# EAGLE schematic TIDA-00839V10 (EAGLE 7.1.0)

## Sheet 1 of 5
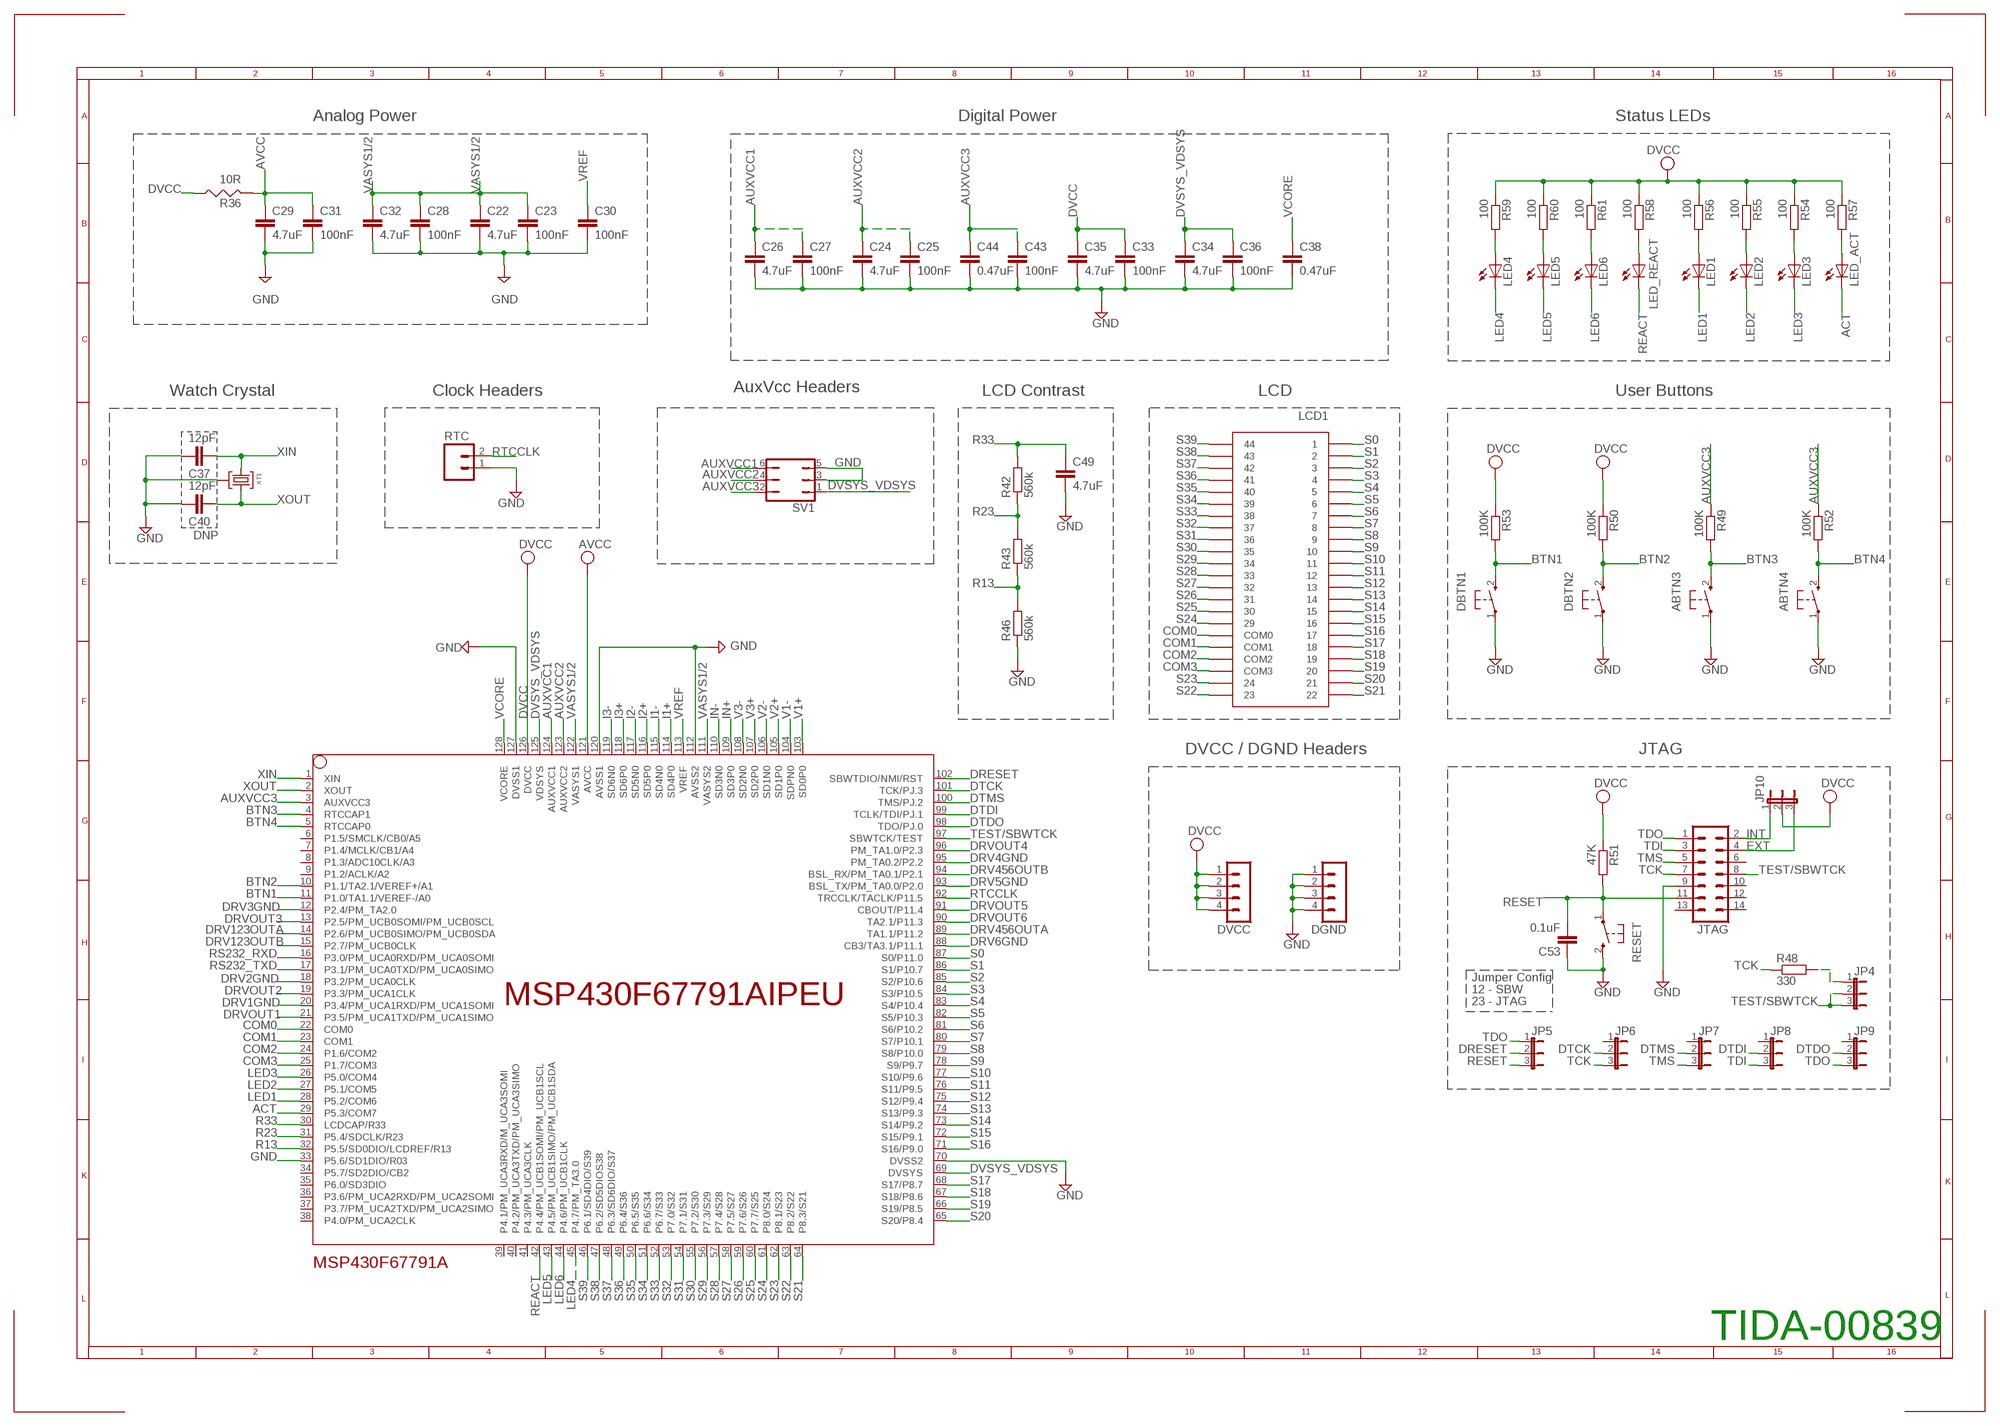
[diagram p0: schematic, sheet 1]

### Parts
ABTN3  PB  [PBTH]
ABTN4  PB  [PBTH]
C22  4.7uF  C-EUC0603  [C0603]
C23  100nF  C-EUC0603  [C0603]
C24  4.7uF  C-EUC0603  [C0603]
C25  100nF  C-EUC0603  [C0603]
C26  4.7uF  C-EUC0603  [C0603]
C27  100nF  C-EUC0603  [C0603]
C28  100nF  C-EUC0603  [C0603]
C29  4.7uF  C-EUC0603  [C0603]
C30  100nF  C-EUC0603  [C0603]
C31  100nF  C-EUC0603  [C0603]
C32  4.7uF  C-EUC0603  [C0603]
C33  100nF  C-EUC0603  [C0603]
C34  4.7uF  C-EUC0603  [C0603]
C35  4.7uF  C-EUC0603  [C0603]
C36  100nF  C-EUC0603  [C0603]
C37  12pF  C-EUC0603  [C0603]
C38  0.47uF  C-EUC0603  [C0603]
C40  12pF  C-EUC0603  [C0603]
C43  100nF  C-EUC0603  [C0603]
C44  0.47uF  C-EUC0603  [C0603]
C49  4.7uF  C-EUC0603  [C0603]
C53  0.1uF  C-EUC0603  [C0603]
DBTN1  PB  [PBTH]
DBTN2  PB  [PBTH]
DGND  MA04-1  [MA04-1]
DVCC  MA04-1  [MA04-1]
JP4  JP2E  [JP2]
JP5  JP2E  [JP2]
JP6  JP2E  [JP2]
JP7  JP2E  [JP2]
JP8  JP2E  [JP2]
JP9  JP2E  [JP2]
JP10  JP2E  [JP2]
JTAG  ML14  [ML14]
LCD1  TI_160SEG_LCD  [TI_160SEG_LCD]
LED1  LED3MM  [LED3MM]
LED2  LED3MM  [LED3MM]
LED3  LED3MM  [LED3MM]
LED4  LED3MM  [LED3MM]
LED5  LED3MM  [LED3MM]
LED6  LED3MM  [LED3MM]
LED_ACT  LED3MM  [LED3MM]
LED_REACT  LED3MM  [LED3MM]
MSP430F67791A  MSP430F6779AIPEU  [PEU128]
R36  10R  RES0805  [R0805]
R42  560k  R-EU_R0603  [R0603]
R43  560k  R-EU_R0603  [R0603]
R46  560k  R-EU_R0603  [R0603]
R48  330  R-EU_R0603  [R0603]
R49  100K  R-EU_R0603  [R0603]
R50  100K  R-EU_R0603  [R0603]
R51  47K  R-EU_R0603  [R0603]
R52  100K  R-EU_R0603  [R0603]
R53  100K  R-EU_R0603  [R0603]
R54  100  R-EU_R0603  [R0603]
R55  100  R-EU_R0603  [R0603]
R56  100  R-EU_R0603  [R0603]
R57  100  R-EU_R0603  [R0603]
R58  100  R-EU_R0603  [R0603]
R59  100  R-EU_R0603  [R0603]
R60  100  R-EU_R0603  [R0603]
R61  100  R-EU_R0603  [R0603]
RESET  PB  [PBTH]
RTC  M02PTH  [1X02]
SV1  JP3Q  [JP3Q]
XT1  CM200T  [CM200T]

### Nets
ACT: LED_ACT.K(C) MSP430F67791A.29(P5.3/COM7) ; also sheet 4
AUXVCC1: C26.1 C27.1 MSP430F67791A.124(AUXVCC1) SV1.6 ; also sheet 5
AUXVCC2: C24.1 C25.1 MSP430F67791A.123(AUXVCC2) SV1.4
AUXVCC3: C43.1 C44.1 MSP430F67791A.3(AUXVCC3) R49.1 R52.1 SV1.2
AVCC: C29.1 C31.1 MSP430F67791A.121(AVCC) R36.2 ; also sheet 2
BTN1: DBTN1.2(S) MSP430F67791A.11(P1.0/TA1.1/VEREF-/A0) R53.2
BTN2: DBTN2.2(S) MSP430F67791A.10(P1.1/TA2.1/VEREF+/A1) R50.2
BTN3: ABTN3.2(S) MSP430F67791A.4(RTCCAP1) R49.2
BTN4: ABTN4.2(S) MSP430F67791A.5(RTCCAP0) R52.2
COM0: LCD1.COM0 MSP430F67791A.22(COM0)
COM1: LCD1.COM1 MSP430F67791A.23(COM1)
COM2: LCD1.COM2 MSP430F67791A.24(P1.6/COM2)
COM3: LCD1.COM3 MSP430F67791A.25(P1.7/COM3)
DRESET: JP5.2 MSP430F67791A.102(SBWTDIO/NMI/RST)
DRV1GND: MSP430F67791A.20(P3.4/PM_UCA1RXD/PM_UCA1SOMI) ; also sheet 5
DRV2GND: MSP430F67791A.18(P3.2/PM_UCA0CLK) ; also sheet 5
DRV3GND: MSP430F67791A.12(P2.4/PM_TA2.0) ; also sheet 5
DRV4GND: MSP430F67791A.95(PM_TA0.2/P2.2) ; also sheet 5
DRV5GND: MSP430F67791A.93(BSL_TX/PM_TA0.0/P2.0) ; also sheet 5
DRV6GND: MSP430F67791A.88(CB3/TA3.1/P11.1) ; also sheet 5
DRV123OUTA: MSP430F67791A.14(P2.6/PM_UCB0SIMO/PM_UCB0SDA) ; also sheet 5
DRV123OUTB: MSP430F67791A.15(P2.7/PM_UCB0CLK) ; also sheet 5
DRV456OUTA: MSP430F67791A.89(TA1.1/P11.2) ; also sheet 5
DRV456OUTB: MSP430F67791A.94(BSL_RX/PM_TA0.1/P2.1) ; also sheet 5
DRVOUT1: MSP430F67791A.21(P3.5/PM_UCA1TXD/PM_UCA1SIMO) ; also sheet 5
DRVOUT2: MSP430F67791A.19(P3.3/PM_UCA1CLK) ; also sheet 5
DRVOUT3: MSP430F67791A.13(P2.5/PM_UCB0SOMI/PM_UCB0SCL) ; also sheet 5
DRVOUT4: MSP430F67791A.96(PM_TA1.0/P2.3) ; also sheet 5
DRVOUT5: MSP430F67791A.91(CBOUT/P11.4) ; also sheet 5
DRVOUT6: MSP430F67791A.90(TA2.1/P11.3) ; also sheet 5
DTCK: JP6.2 MSP430F67791A.101(TCK/PJ.3)
DTDI: JP8.2 MSP430F67791A.99(TCLK/TDI/PJ.1)
DTDO: JP9.2 MSP430F67791A.98(TDO/PJ.0)
DTMS: JP7.2 MSP430F67791A.100(TMS/PJ.2)
DVCC: C33.1 C35.1 DVCC.1 DVCC.2 DVCC.3 DVCC.4 JP10.2 MSP430F67791A.126(DVCC) R36.1 R50.1 R51.1 R53.1 R54.1 R55.1 R56.1 R57.1 R58.1 R59.1 R60.1 R61.1 ; also sheet 3,4,5
DVSYS_VDSYS: C34.1 C36.1 MSP430F67791A.69(DVSYS) MSP430F67791A.125(VDSYS) SV1.1 ; also sheet 5
EXT: JP10.3 JTAG.4
GND: ABTN3.1(P) ABTN4.1(P) C22.2 C23.2 C24.2 C25.2 C26.2 C27.2 C28.2 C29.2 C30.2 C31.2 C32.2 C33.2 C34.2 C35.2 C36.2 C37.2 C38.2 C40.2 C43.2 C44.2 C49.2 C53.1 DBTN1.1(P) DBTN2.1(P) DGND.1 DGND.2 DGND.3 DGND.4 JTAG.9 MSP430F67791A.33(P5.6/SD1DIO/R03) MSP430F67791A.70(DVSS2) MSP430F67791A.112(AVSS2) MSP430F67791A.120(AVSS1) MSP430F67791A.127(DVSS1) R46.1 RESET.2(S) RTC.1 SV1.3 SV1.5 XT1.P3 ; also sheet 2,3,4,5
I1+: MSP430F67791A.114(SD4P0) ; also sheet 2
I1-: MSP430F67791A.115(SD4N0) ; also sheet 2
I2+: MSP430F67791A.116(SD5P0) ; also sheet 2
I2-: MSP430F67791A.117(SD5N0) ; also sheet 2
I3+: MSP430F67791A.118(SD6P0) ; also sheet 2
I3-: MSP430F67791A.119(SD6N0) ; also sheet 2
IN+: MSP430F67791A.109(SD3P0) ; also sheet 2
IN-: MSP430F67791A.110(SD3N0) ; also sheet 2
INT: JP10.1 JTAG.2
LED1: LED1.K(C) MSP430F67791A.28(P5.2/COM6)
LED2: LED2.K(C) MSP430F67791A.27(P5.1/COM5)
LED3: LED3.K(C) MSP430F67791A.26(P5.0/COM4)
LED4: LED4.K(C) MSP430F67791A.45(P4.7/PM_TA3.0)
LED5: LED5.K(C) MSP430F67791A.43(P4.5/PM_UCB1SIMO/PM_UCB1SDA)
LED6: LED6.K(C) MSP430F67791A.44(P4.6/PM_UCB1CLK)
N$4: LED1.A R56.2
N$7: LED2.A R55.2
N$10: JP4.1 R48.2
N$21: LED4.A R59.2
N$27: LED5.A R60.2
N$30: LED3.A R54.2
N$36: LED6.A R61.2
N$44: LED_REACT.A R58.2
N$46: LED_ACT.A R57.2
R13: MSP430F67791A.32(P5.5/SD0DIO/LCDREF/R13) R43.1 R46.2
R23: MSP430F67791A.31(P5.4/SDCLK/R23) R42.1 R43.2
R33: C49.1 MSP430F67791A.30(LCDCAP/R33) R42.2
REACT: LED_REACT.K(C) MSP430F67791A.42(P4.4/PM_UCB1SOMI/PM_UCB1SCL) ; also sheet 4
RESET: C53.2 JP5.3 JTAG.11 R51.2 RESET.1(P)
RS232_RXD: MSP430F67791A.16(P3.0/PM_UCA0RXD/PM_UCA0SOMI) ; also sheet 4
RS232_TXD: MSP430F67791A.17(P3.1/PM_UCA0TXD/PM_UCA0SIMO) ; also sheet 4
RTCCLK: MSP430F67791A.92(TRCCLK/TACLK/P11.5) RTC.2
S0: LCD1.1 MSP430F67791A.87(S0/P11.0)
S1: LCD1.2 MSP430F67791A.86(S1/P10.7)
S2: LCD1.3 MSP430F67791A.85(S2/P10.6)
S3: LCD1.4 MSP430F67791A.84(S3/P10.5)
S4: LCD1.5 MSP430F67791A.83(S4/P10.4)
S5: LCD1.6 MSP430F67791A.82(S5/P10.3)
S6: LCD1.7 MSP430F67791A.81(S6/P10.2)
S7: LCD1.8 MSP430F67791A.80(S7/P10.1)
S8: LCD1.9 MSP430F67791A.79(S8/P10.0)
S9: LCD1.10 MSP430F67791A.78(S9/P9.7)
S10: LCD1.11 MSP430F67791A.77(S10/P9.6)
S11: LCD1.12 MSP430F67791A.76(S11/P9.5)
S12: LCD1.13 MSP430F67791A.75(S12/P9.4)
S13: LCD1.14 MSP430F67791A.74(S13/P9.3)
S14: LCD1.15 MSP430F67791A.73(S14/P9.2)
S15: LCD1.16 MSP430F67791A.72(S15/P9.1)
S16: LCD1.17 MSP430F67791A.71(S16/P9.0)
S17: LCD1.18 MSP430F67791A.68(S17/P8.7)
S18: LCD1.19 MSP430F67791A.67(S18/P8.6)
S19: LCD1.20 MSP430F67791A.66(S19/P8.5)
S20: LCD1.21 MSP430F67791A.65(S20/P8.4)
S21: LCD1.22 MSP430F67791A.64(P8.3/S21)
S22: LCD1.23 MSP430F67791A.63(P8.2/S22)
S23: LCD1.24 MSP430F67791A.62(P8.1/S23)
S24: LCD1.29 MSP430F67791A.61(P8.0/S24)
S25: LCD1.30 MSP430F67791A.60(P7.7/S25)
S26: LCD1.31 MSP430F67791A.59(P7.6/S26)
S27: LCD1.32 MSP430F67791A.58(P7.5/S27)
S28: LCD1.33 MSP430F67791A.57(P7.4/S28)
S29: LCD1.34 MSP430F67791A.56(P7.3/S29)
S30: LCD1.35 MSP430F67791A.55(P7.2/S30)
S31: LCD1.36 MSP430F67791A.54(P7.1/S31)
S32: LCD1.37 MSP430F67791A.53(P7.0/S32)
S33: LCD1.38 MSP430F67791A.52(P6.7/S33)
S34: LCD1.39 MSP430F67791A.51(P6.6/S34)
S35: LCD1.40 MSP430F67791A.50(P6.5/S35)
S36: LCD1.41 MSP430F67791A.49(P6.4/S36)
S37: LCD1.42 MSP430F67791A.48(P6.3/SD6DIO/S37)
S38: LCD1.43 MSP430F67791A.47(P6.2/SD5DIOS38)
S39: LCD1.44 MSP430F67791A.46(P6.1/SD4DIO/S39)
TCK: JP6.3 JTAG.7 R48.1
TDI: JP8.3 JTAG.3
TDO: JP5.1 JP9.3 JTAG.1
TEST/SBWTCK: JP4.2 JP4.3 JTAG.8 MSP430F67791A.97(SBWTCK/TEST)
TMS: JP7.3 JTAG.5
V1+: MSP430F67791A.103(SD0P0) ; also sheet 2
V1-: MSP430F67791A.104(SDPN0) ; also sheet 2
V2+: MSP430F67791A.105(SD1P0) ; also sheet 2
V2-: MSP430F67791A.106(SD1N0) ; also sheet 2
V3+: MSP430F67791A.107(SD2P0) ; also sheet 2
V3-: MSP430F67791A.108(SD2N0) ; also sheet 2
VASYS1/2: C22.1 C23.1 C28.1 C32.1 MSP430F67791A.111(VASYS2) MSP430F67791A.122(VASYS1)
VCORE: C38.1 MSP430F67791A.128(VCORE)
VREF: C30.1 MSP430F67791A.113(VREF)
XIN: C37.1 MSP430F67791A.1(XIN) XT1.P2
XOUT: C40.1 MSP430F67791A.2(XOUT) XT1.P1
Unconnected: JP6.1 JP7.1 JP8.1 JP9.1 JTAG.6 JTAG.10 JTAG.12 JTAG.13 JTAG.14 MSP430F67791A.6(P1.5/SMCLK/CB0/A5) MSP430F67791A.7(P1.4/MCLK/CB1/A4) MSP430F67791A.8(P1.3/ADC10CLK/A3) MSP430F67791A.9(P1.2/ACLK/A2) MSP430F67791A.34(P5.7/SD2DIO/CB2) MSP430F67791A.35(P6.0/SD3DIO) MSP430F67791A.36(P3.6/PM_UCA2RXD/PM_UCA2SOMI) MSP430F67791A.37(P3.7/PM_UCA2TXD/PM_UCA2SIMO) MSP430F67791A.38(P4.0/PM_UCA2CLK) MSP430F67791A.39(P4.1/PM_UCA3RXD/M_UCA3SOMI) MSP430F67791A.40(P4.2/PM_UCA3TXD/PM_UCA3SIMO) MSP430F67791A.41(P4.3/PM_UCA3CLK)

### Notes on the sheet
- Analog Power | Digital Power | Status LEDs
- Watch Crystal | Clock Headers | AuxVcc Headers | LCD Contrast | LCD | User Buttons
- DNP
- DVCC / DGND Headers | JTAG
- Jumper Config
- 12 - SBW
- 23 - JTAG
- TIDA-00839

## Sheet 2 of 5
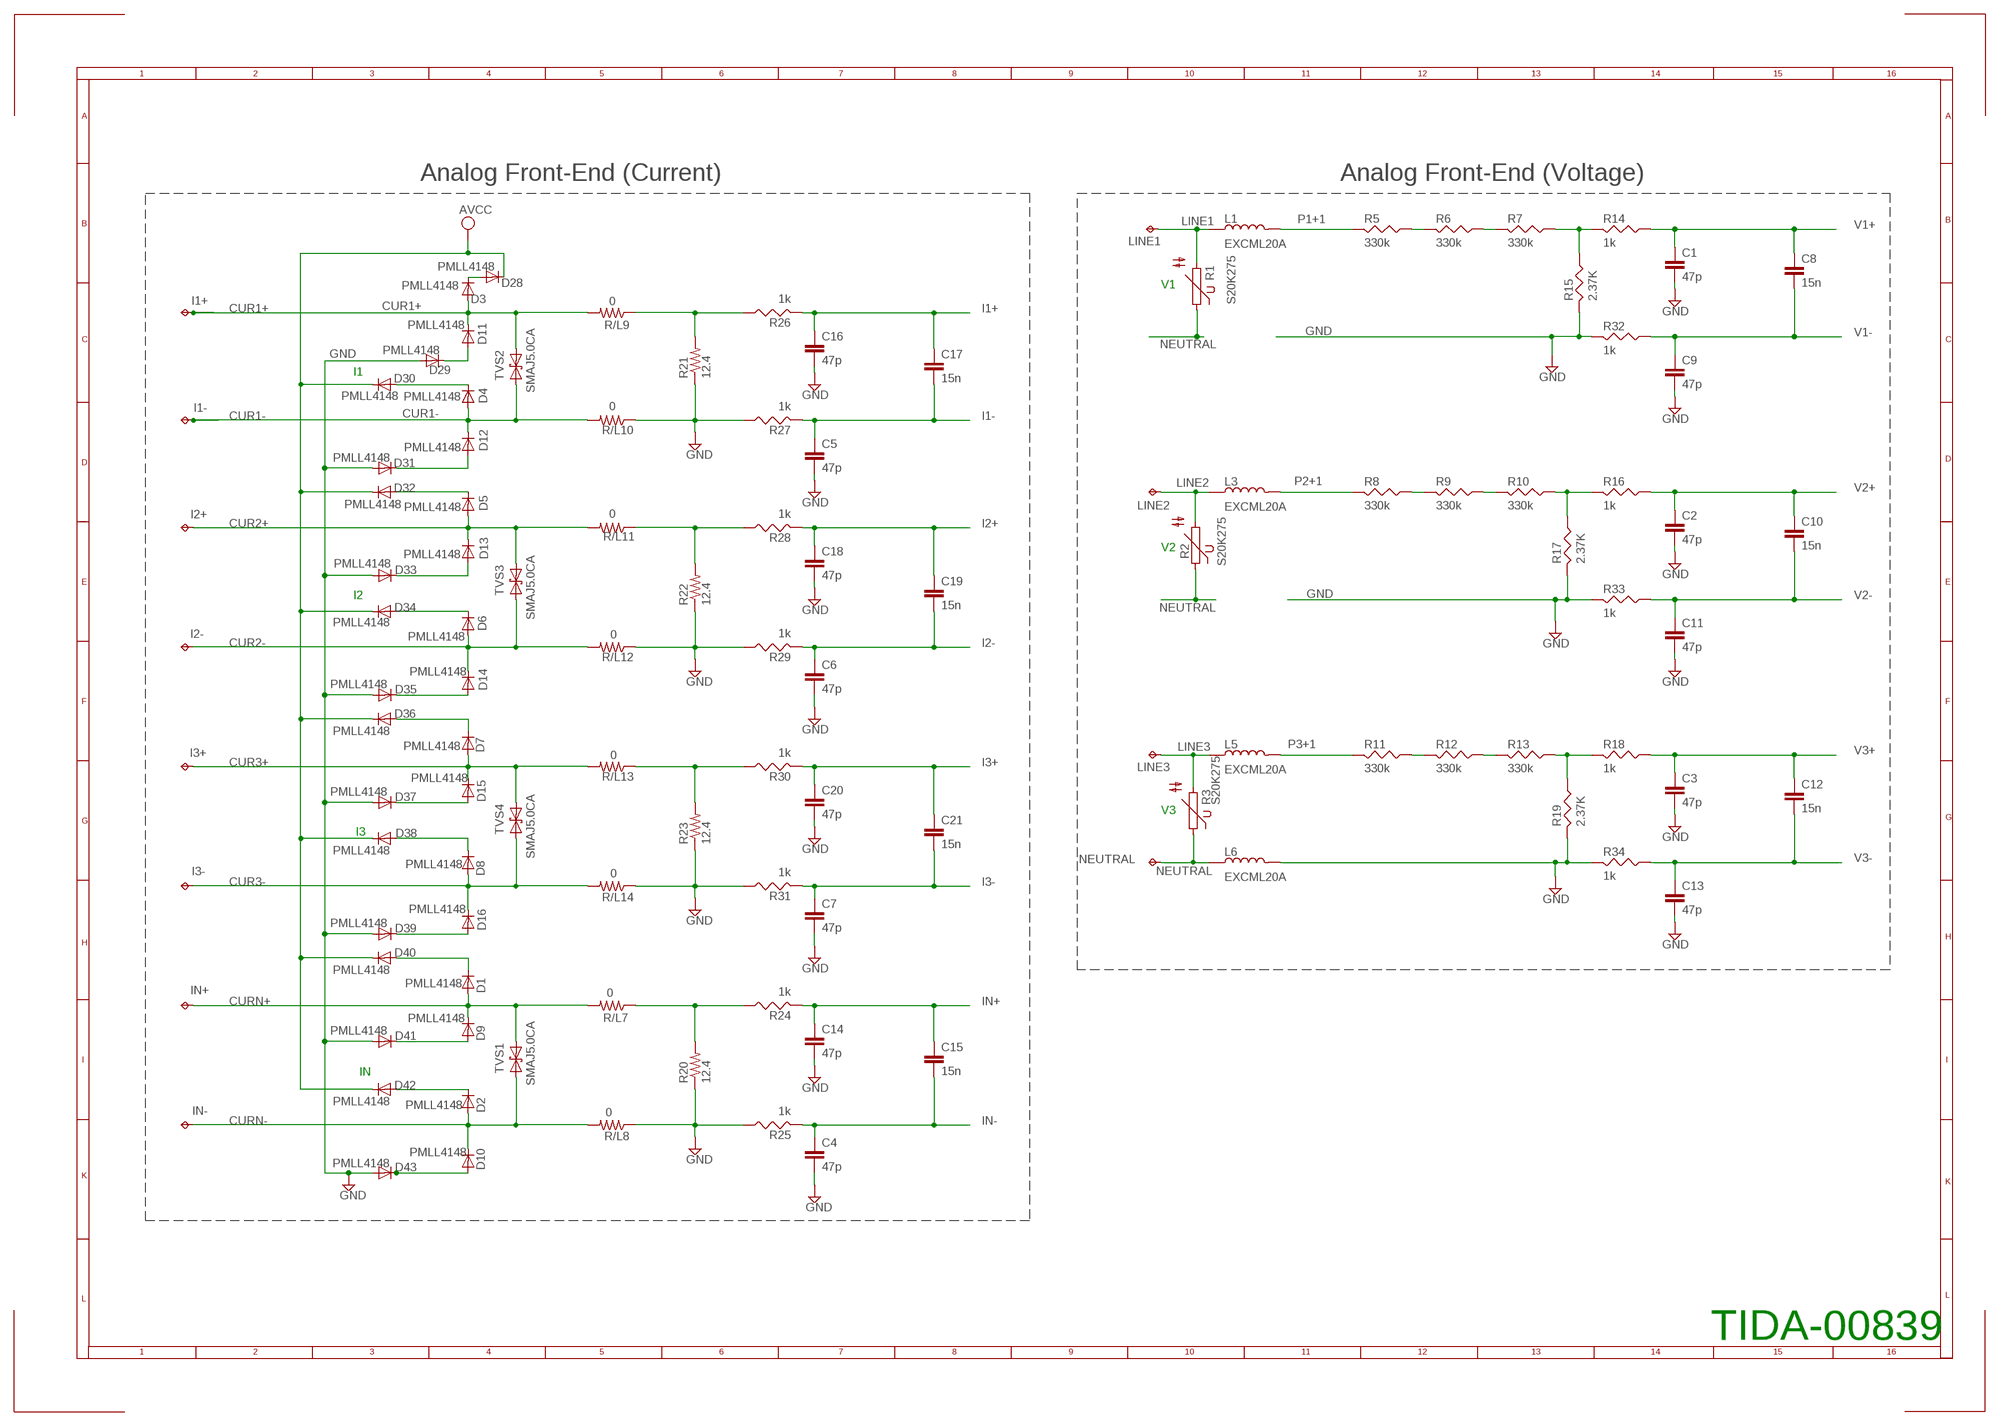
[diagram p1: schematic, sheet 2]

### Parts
C1  47p  C-EUC0805  [C0805]
C2  47p  C-EUC0805  [C0805]
C3  47p  C-EUC0805  [C0805]
C4  47p  C-EUC0805  [C0805]
C5  47p  C-EUC0805  [C0805]
C6  47p  C-EUC0805  [C0805]
C7  47p  C-EUC0805  [C0805]
C8  15n  C-EUC0805  [C0805]
C9  47p  C-EUC0805  [C0805]
C10  15n  C-EUC0805  [C0805]
C11  47p  C-EUC0805  [C0805]
C12  15n  C-EUC0805  [C0805]
C13  47p  C-EUC0805  [C0805]
C14  47p  C-EUC0805  [C0805]
C15  15n  C-EUC0805  [C0805]
C16  47p  C-EUC0805  [C0805]
C17  15n  C-EUC0805  [C0805]
C18  47p  C-EUC0805  [C0805]
C19  15n  C-EUC0805  [C0805]
C20  47p  C-EUC0805  [C0805]
C21  15n  C-EUC0805  [C0805]
D1  PMLL4148  [SOD80C]
D2  PMLL4148  [SOD80C]
D3  PMLL4148  [SOD80C]
D4  PMLL4148  [SOD80C]
D5  PMLL4148  [SOD80C]
D6  PMLL4148  [SOD80C]
D7  PMLL4148  [SOD80C]
D8  PMLL4148  [SOD80C]
D9  PMLL4148  [SOD80C]
D10  PMLL4148  [SOD80C]
D11  PMLL4148  [SOD80C]
D12  PMLL4148  [SOD80C]
D13  PMLL4148  [SOD80C]
D14  PMLL4148  [SOD80C]
D15  PMLL4148  [SOD80C]
D16  PMLL4148  [SOD80C]
D28  PMLL4148  [SOD80C]
D29  PMLL4148  [SOD80C]
D30  PMLL4148  [SOD80C]
D31  PMLL4148  [SOD80C]
D32  PMLL4148  [SOD80C]
D33  PMLL4148  [SOD80C]
D34  PMLL4148  [SOD80C]
D35  PMLL4148  [SOD80C]
D36  PMLL4148  [SOD80C]
D37  PMLL4148  [SOD80C]
D38  PMLL4148  [SOD80C]
D39  PMLL4148  [SOD80C]
D40  PMLL4148  [SOD80C]
D41  PMLL4148  [SOD80C]
D42  PMLL4148  [SOD80C]
D43  PMLL4148  [SOD80C]
I1+  TPPAD1-20  [P1-20]
I1-  TPPAD1-20  [P1-20]
I2+  TPPAD1-20  [P1-20]
I2-  TPPAD1-20  [P1-20]
I3+  TPPAD1-20  [P1-20]
I3-  TPPAD1-20  [P1-20]
IN+  TPPAD1-20  [P1-20]
IN-  TPPAD1-20  [P1-20]
L1  EXCML20A  EXCELSA390805  [R0805]
L3  EXCML20A  EXCELSA390805  [R0805]
L5  EXCML20A  EXCELSA390805  [R0805]
L6  EXCML20A  EXCELSA390805  [R0805]
LINE1  TPPAD1-20  [P1-20]
LINE2  TPPAD1-20  [P1-20]
LINE3  TPPAD1-20  [P1-20]
NEUTRAL  TPPAD1-20  [P1-20]
R1  S20K275  [S20K275]
R2  S20K275  [S20K275]
R3  S20K275  [S20K275]
R5  330k  RES0805  [R0805]
R6  330k  RES0805  [R0805]
R7  330k  RES0805  [R0805]
R8  330k  RES0805  [R0805]
R9  330k  RES0805  [R0805]
R10  330k  RES0805  [R0805]
R11  330k  RES0805  [R0805]
R12  330k  RES0805  [R0805]
R13  330k  RES0805  [R0805]
R14  1k  RES0805  [R0805]
R15  2.37K  RES0805  [R0805]
R16  1k  RES0805  [R0805]
R17  2.37K  RES0805  [R0805]
R18  1k  RES0805  [R0805]
R19  2.37K  RES0805  [R0805]
R20  12.4  R-US_R0805  [R0805]
R21  12.4  R-US_R0805  [R0805]
R22  12.4  R-US_R0805  [R0805]
R23  12.4  R-US_R0805  [R0805]
R24  1k  RES0805  [R0805]
R25  1k  RES0805  [R0805]
R26  1k  RES0805  [R0805]
R27  1k  RES0805  [R0805]
R28  1k  RES0805  [R0805]
R29  1k  RES0805  [R0805]
R30  1k  RES0805  [R0805]
R31  1k  RES0805  [R0805]
R32  1k  RES0805  [R0805]
R33  1k  RES0805  [R0805]
R34  1k  RES0805  [R0805]
R/L7  0  R-US_R0805  [R0805]
R/L8  0  R-US_R0805  [R0805]
R/L9  0  R-US_R0805  [R0805]
R/L10  0  R-US_R0805  [R0805]
R/L11  0  R-US_R0805  [R0805]
R/L12  0  R-US_R0805  [R0805]
R/L13  0  R-US_R0805  [R0805]
R/L14  0  R-US_R0805  [R0805]
TVS1  SMAJ5.0CA  [DO214AC]
TVS2  SMAJ5.0CA  [DO214AC]
TVS3  SMAJ5.0CA  [DO214AC]
TVS4  SMAJ5.0CA  [DO214AC]

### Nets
AVCC: D28.C D30.C D32.C D34.C D36.C D38.C D40.C D42.C ; also sheet 1
CUR1+: D3.A D11.C I1+.TP R/L9.2 TVS2.C(K)
CUR1-: D4.A D12.C I1-.TP R/L10.2 TVS2.A
CUR2+: D5.A D13.C I2+.TP R/L11.2 TVS3.C(K)
CUR2-: D6.A D14.C I2-.TP R/L12.2 TVS3.A
CUR3+: D7.A D15.C I3+.TP R/L13.2 TVS4.C(K)
CUR3-: D8.A D16.C I3-.TP R/L14.2 TVS4.A
CURN+: D1.A D9.C IN+.TP R/L7.2 TVS1.C(K)
CURN-: D2.A D10.C IN-.TP R/L8.2 TVS1.A
GND: C1.2 C2.2 C3.2 C4.2 C5.2 C6.2 C7.2 C9.2 C11.2 C13.2 C14.2 C16.2 C18.2 C20.2 D29.A D31.A D33.A D35.A D37.A D39.A D41.A D43.A L6.2 R15.2 R17.2 R19.2 R20.1 R21.1 R22.1 R23.1 R25.1 R27.1 R29.1 R31.1 R32.2 R33.2 R34.2 R/L8.1 R/L10.1 R/L12.1 R/L14.1 ; also sheet 1,3,4,5
I1+: C16.1 C17.1 R26.2 ; also sheet 1
I1-: C5.1 C17.2 R27.2 ; also sheet 1
I2+: C18.1 C19.1 R28.2 ; also sheet 1
I2-: C6.1 C19.2 R29.2 ; also sheet 1
I3+: C20.1 C21.1 R30.2 ; also sheet 1
I3-: C7.1 C21.2 R31.2 ; also sheet 1
IN+: C14.1 C15.1 R24.2 ; also sheet 1
IN-: C4.1 C15.2 R25.2 ; also sheet 1
LINE1: L1.1 LINE1.TP R1.2
LINE2: L3.1 LINE2.TP R2.2
LINE3: L5.1 LINE3.TP R3.2
N$6: R20.2 R24.1 R/L7.1
N$8: R5.1 R6.2
N$13: R6.1 R7.2
N$14: R7.1 R14.2 R15.1
N$15: R8.1 R9.2
N$16: R9.1 R10.2
N$19: R10.1 R16.2 R17.1
N$20: D3.C D28.A
N$23: D11.A D29.C
N$25: R23.2 R30.1 R/L13.1
N$29: R11.1 R12.2
N$31: R22.2 R28.1 R/L11.1
N$32: R21.2 R26.1 R/L9.1
N$33: R12.1 R13.2
N$34: R13.1 R18.2 R19.1
N$39: D4.C D30.A
N$40: D12.A D31.C
N$42: D5.C D32.A
N$54: D13.A D33.C
N$62: D6.C D34.A
N$63: D14.A D35.C
N$64: D7.C D36.A
N$66: D15.A D37.C
N$70: D8.C D38.A
N$73: D16.A D39.C
N$74: D1.C D40.A
N$75: D9.A D41.C
N$76: D2.C D42.A
N$77: D10.A D43.C
NEUTRAL: L6.1 NEUTRAL.TP R1.1 R2.1 R3.1 ; also sheet 3
P1+1: L1.2 R5.2 ; also sheet 3
P2+1: L3.2 R8.2 ; also sheet 3
P3+1: L5.2 R11.2 ; also sheet 3
V1+: C1.1 C8.1 R14.1 ; also sheet 1
V1-: C8.2 C9.1 R32.1 ; also sheet 1
V2+: C2.1 C10.1 R16.1 ; also sheet 1
V2-: C10.2 C11.1 R33.1 ; also sheet 1
V3+: C3.1 C12.1 R18.1 ; also sheet 1
V3-: C12.2 C13.1 R34.1 ; also sheet 1

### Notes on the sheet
- Analog Front-End (Current) | Analog Front-End (Voltage)
- V1
- I1
- V2
- I2
- V3
- I3
- IN
- TIDA-00839

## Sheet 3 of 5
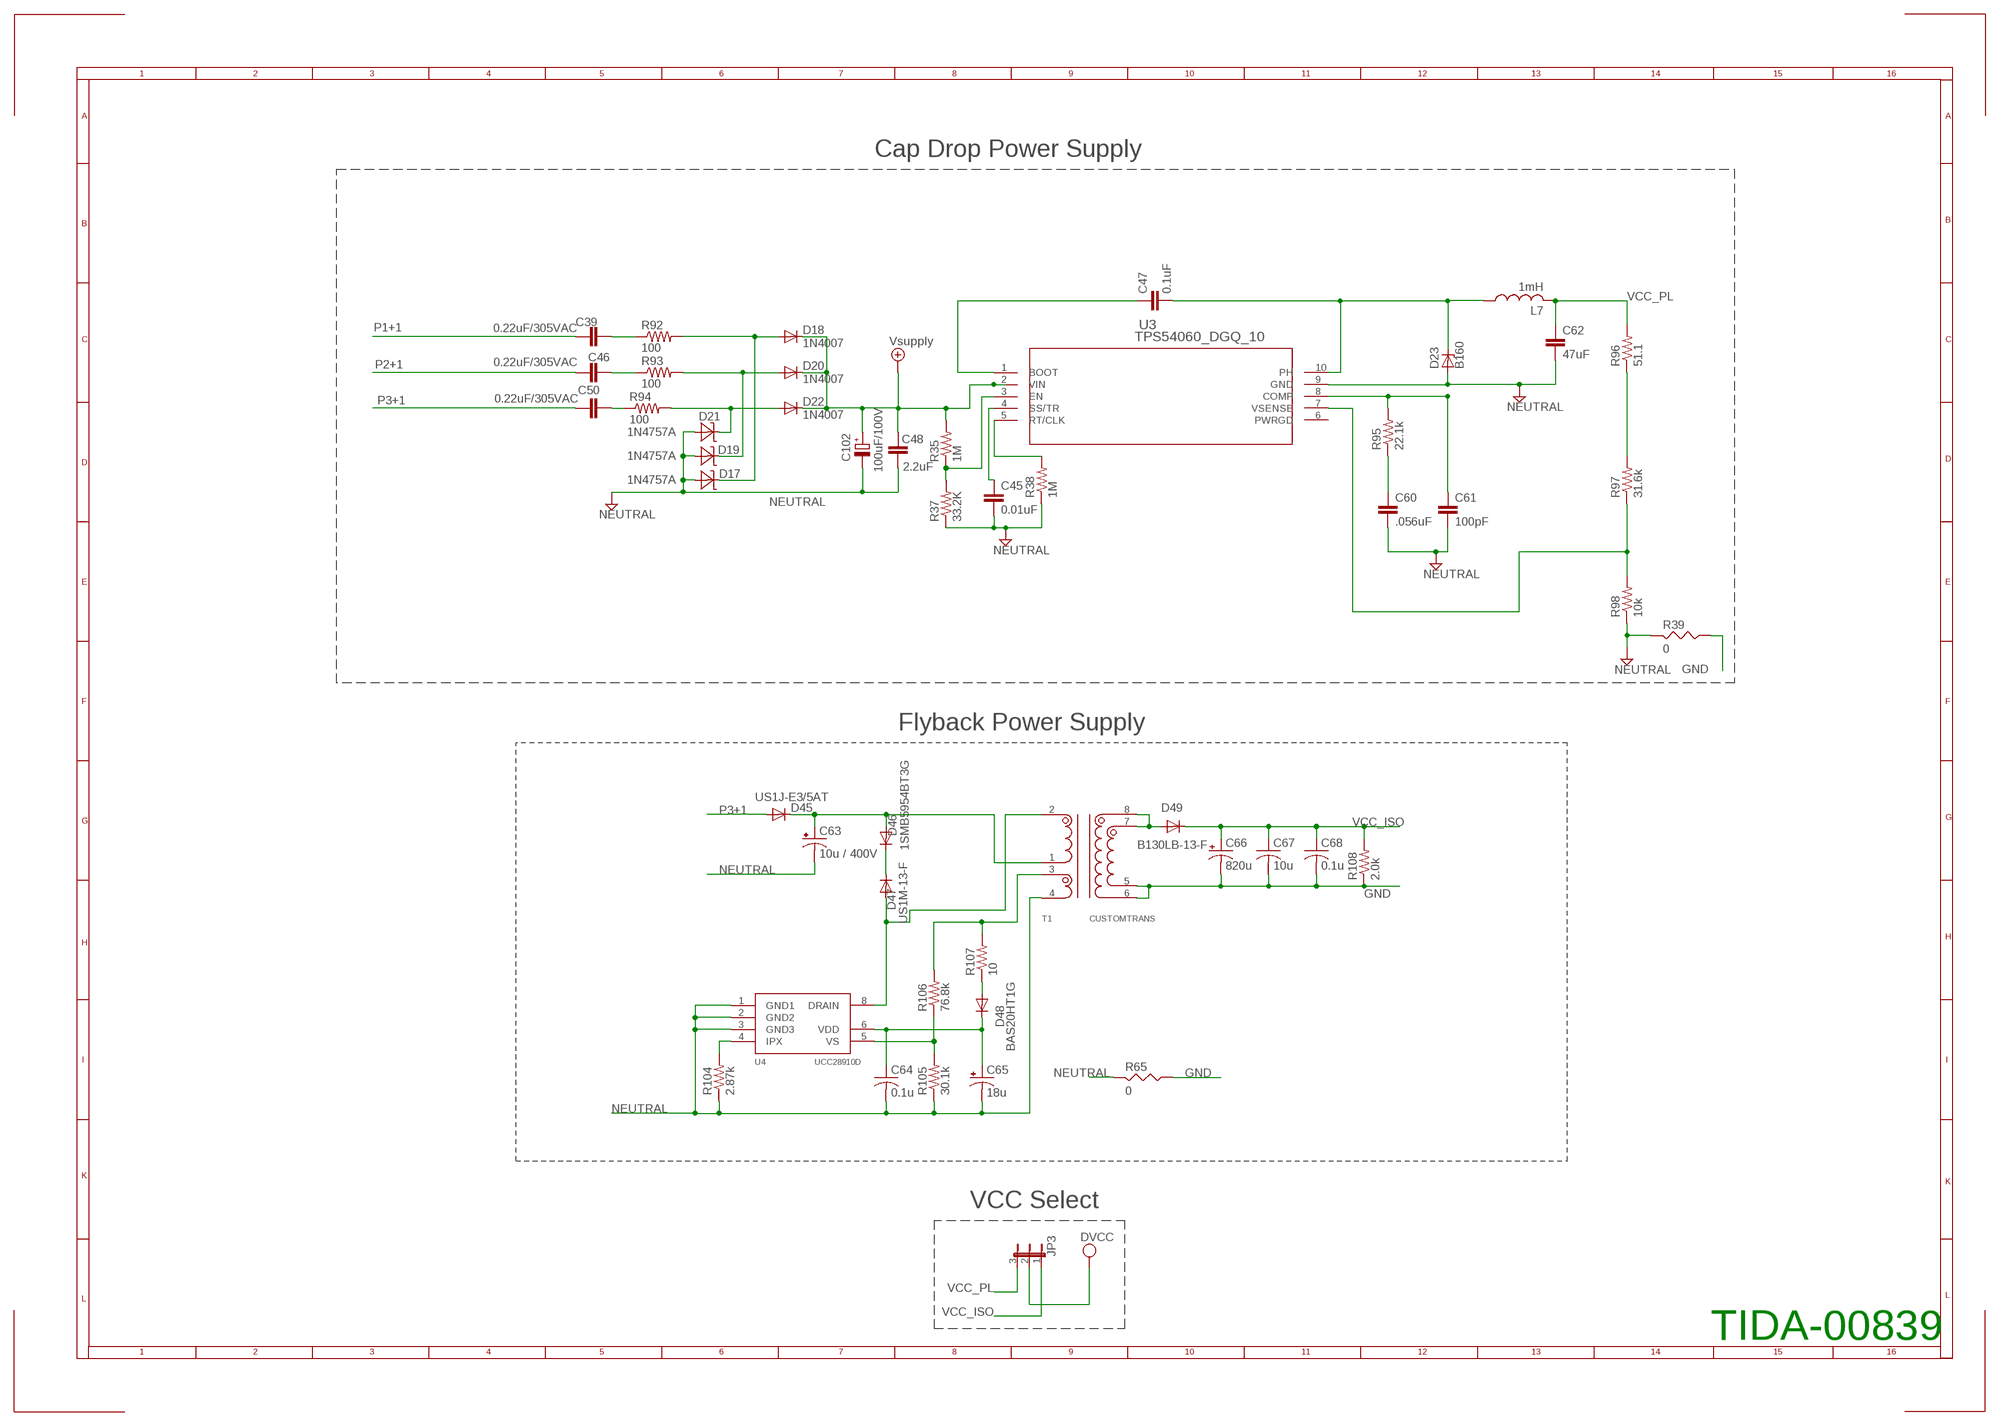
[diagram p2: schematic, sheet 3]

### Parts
C39  0.22uF/305VAC  C15/8  [C15B8]
C45  0.01uF  C-EUC0603  [C0603]
C46  0.22uF/305VAC  C15/8  [C15B8]
C47  0.1uF  C-EUC0603  [C0603]
C48  2.2uF  C-EUC1210  [C1210]
C50  0.22uF/305VAC  C15/8  [C15B8]
C60  .056uF  C-EUC0603  [C0603]
C61  100pF  C-EUC0603  [C0603]
C62  47uF  C-EUC1210  [C1210]
C63  10u / 400V  CPOL-USE5-10.5  [E5-10,5]
C64  0.1u  C-USC0603  [C0603]
C65  18u  CPOL-USE5-5  [E5-5]
C66  820u  CPOL-USE3.5-8  [E3,5-8]
C67  10u  C-USC1210  [C1210]
C68  0.1u  C-USC0805  [C0805]
C102  100uF/100V  CPOL-EUE5-10.5  [E5-10,5]
D17  1N4757A  [DO41Z10]
D18  1N4007  [DO41-10]
D19  1N4757A  [DO41Z10]
D20  1N4007  [DO41-10]
D21  1N4757A  [DO41Z10]
D22  1N4007  [DO41-10]
D23  B160  ZENER-DIODESMB  [SMB]
D45  US1J-E3/5AT  DIODE-DO-214AC  [DO-214AC]
D46  1SMB5954BT3G  DIODE-DO-214AC  [DO-214AC]
D47  US1M-13-F  DIODE-DO-214AC  [DO-214AC]
D48  BAS20HT1G  DIODE-SOD323-R  [SOD323-R]
D49  B130LB-13-F  DIODE-DO214AA  [DO214AA]
JP3  JP2E  [JP2]
L7  1mH  L-USMSS1038-105  [INDUCTOR_POWER_SUPPLY_6779]
R35  1M  R-US_R0603  [R0603]
R37  33.2K  R-US_R0603  [R0603]
R38  1M  R-US_R0603  [R0603]
R39  0  RES0805  [R0805]
R65  0  RES0805  [R0805]
R92  100  R-US_0414/15  [0414/15]
R93  100  R-US_0414/15  [0414/15]
R94  100  R-US_0414/15  [0414/15]
R95  22.1k  R-US_R0603  [R0603]
R96  51.1  R-US_R0603  [R0603]
R97  31.6k  R-US_R0603  [R0603]
R98  10k  R-US_R0603  [R0603]
R104  2.87k  R-US_R0603  [R0603]
R105  30.1k  R-US_R0603  [R0603]
R106  76.8k  R-US_R0603  [R0603]
R107  10  R-US_R0603  [R0603]
R108  2.0k  R-US_R0603  [R0603]
T1  CUSTOMTRANS  [TRANS]
U3  TPS54060_DGQ_10  [DGQ10_1P88X1P57]
U4  UCC28910D  [SOIC(D)]

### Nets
DVCC: JP3.2 ; also sheet 1,4,5
GND: C66.- C67.2 C68.2 R39.1 R65.1 R108.1 T1.5 T1.6 ; also sheet 1,2,4,5
N$17: R38.2 U3.5(RT/CLK)
N$18: D17.C D18.A R92.2
N$37: C45.1 U3.4(SS/TR)
N$38: R35.1 R37.2 U3.3(EN)
N$47: D19.C D20.A R93.2
N$78: C47.1 U3.1(BOOT)
N$80: C47.2 D23.C L7.1 U3.10(PH)
N$82: C60.1 R95.1
N$84: C39.2 R92.1
N$89: C46.2 R93.1
N$90: C50.2 R94.1
N$91: C63.+ D45.C D46.A T1.1
N$92: C61.1 R95.2 U3.8(COMP)
N$93: R96.1 R97.2
N$94: D21.C D22.A R94.2
N$95: R97.1 R98.2 U3.7(VSENSE)
N$96: D46.C D47.C
N$97: R104.2 U4.4(IPX)
N$98: D47.A T1.2 U4.8(DRAIN)
N$99: C64.1 C65.+ D48.C U4.6(VDD)
N$100: R105.2 R106.1 U4.5(VS)
N$101: D48.A R107.1
N$102: R106.2 R107.2 T1.3
N$103: D49.A T1.7 T1.8
NEUTRAL: C45.2 C48.2 C60.2 C61.2 C62.2 C63.- C64.2 C65.- C102.- D17.A D19.A D21.A D23.A R37.1 R38.1 R39.2 R65.2 R98.1 R104.1 R105.1 T1.4 U3.9(GND) U4.1(GND1) U4.2(GND2) U4.3(GND3) ; also sheet 2
P1+1: C39.1 ; also sheet 2
P2+1: C46.1 ; also sheet 2
P3+1: C50.1 D45.A ; also sheet 2
VCC_ISO: C66.+ C67.1 C68.1 D49.C JP3.1 R108.2
VCC_PL: C62.1 JP3.3 L7.2 R96.2
VSUPPLY: C48.1 C102.+ D18.C D20.C D22.C R35.2 U3.2(VIN) ; supply symbol labelled Vsupply
Unconnected: U3.6(PWRGD)

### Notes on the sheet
- Cap Drop Power Supply
- Flyback Power Supply
- VCC Select
- TIDA-00839

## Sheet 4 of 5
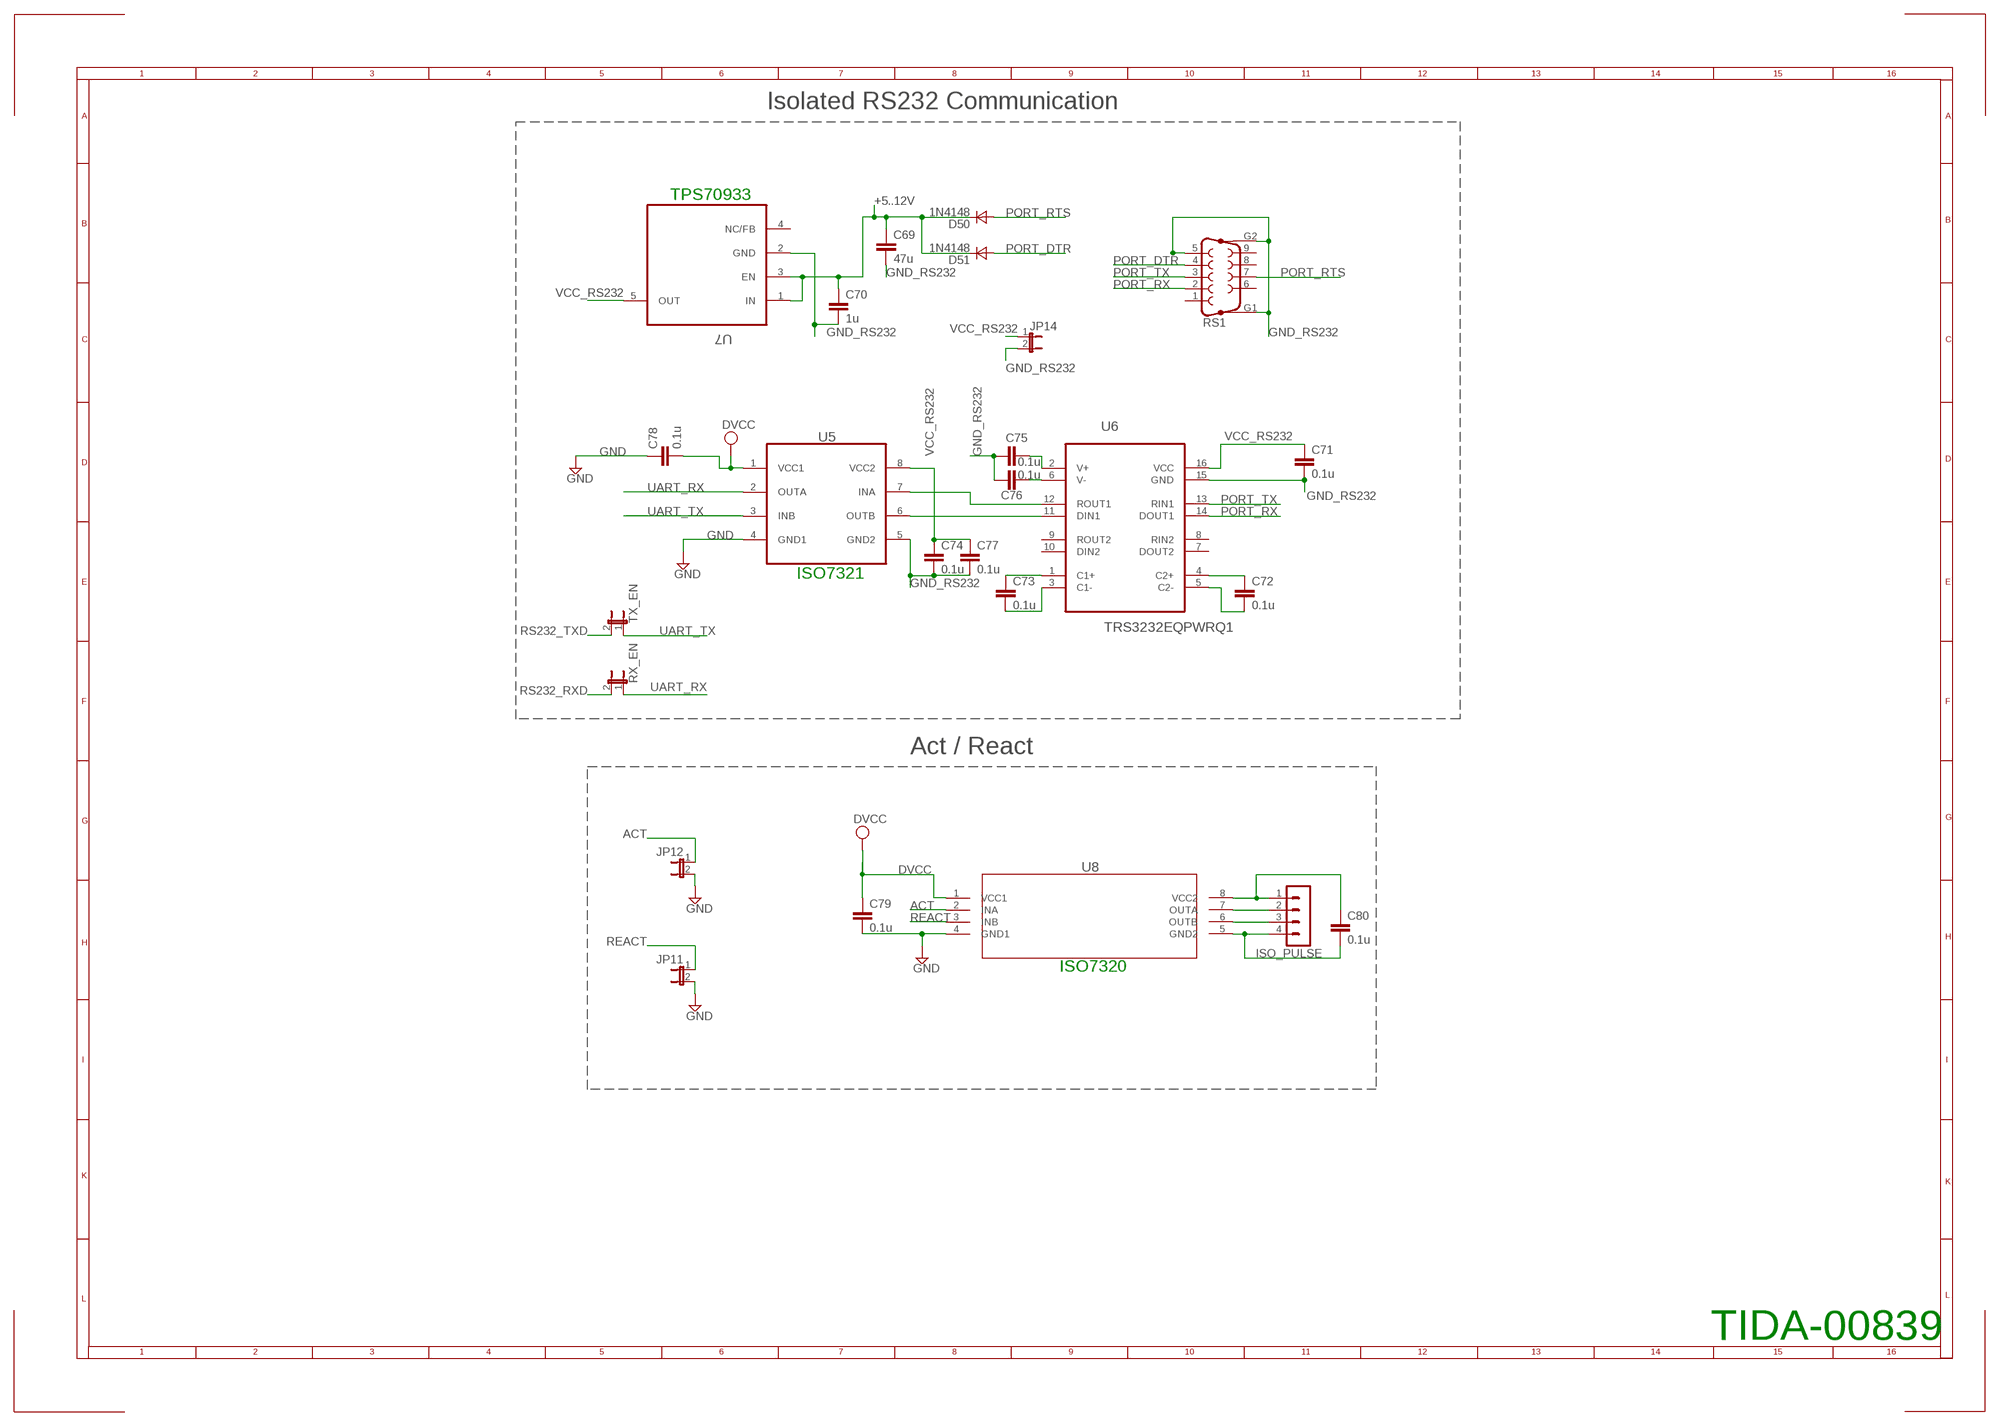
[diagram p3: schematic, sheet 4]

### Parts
C69  47u  C-EUC1206K  [C1206K]
C70  1u  C-EUC0603  [C0603]
C71  0.1u  C-EUC0603  [C0603]
C72  0.1u  C-EUC0603  [C0603]
C73  0.1u  C-EUC0603  [C0603]
C74  0.1u  C-EUC0603  [C0603]
C75  0.1u  C-EUC0603  [C0603]
C76  0.1u  C-EUC0603  [C0603]
C77  0.1u  C-EUC0603  [C0603]
C78  0.1u  C-EUC0603  [C0603]
C79  0.1u  C-EUC0603  [C0603]
C80  0.1u  C-EUC0603  [C0603]
D50  1N4148  DSOD323  [SOD323]
D51  1N4148  DSOD323  [SOD323]
ISO_PULSE  MA04-1  [MA04-1]
JP11  JP1E  [JP1]
JP12  JP1E  [JP1]
JP14  JP1E  [JP1]
RS1  F09VP  [F09VP]
RX_EN  JP1E  [JP1]
TX_EN  JP1E  [JP1]
U5  ISO7421D  [SOIC127P600X175-8N]
U6  TRS3232EQPWRQ1  [SOP65P640X120-16N]
U7  TPS76333DBVT  [SOT95P280X145-5N]
U8  ISO7420_D_8  [D8]

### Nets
+5..12V: C69.1 C70.1 D50.1(C) D51.1(C) U7.1(IN) U7.3(EN)
ACT: JP12.1 U8.2(INA) ; also sheet 1
DVCC: C78.2 C79.1 U5.1(VCC1) U8.1(VCC1) ; also sheet 1,3,5
GND: C78.1 C79.2 JP11.2 JP12.2 U5.4(GND1) U8.4(GND1) ; also sheet 1,2,3,5
GND_RS232: C69.2 C70.2 C71.2 C74.2 C75.1 C76.1 C77.2 JP14.2 RS1.5 RS1.G1 RS1.G2 U5.5(GND2) U6.15(GND) U7.2(GND)
N$104: C72.1 U6.4(C2+)
N$105: C72.2 U6.5(C2-)
N$106: C73.1 U6.1(C1+)
N$107: C73.2 U6.3(C1-)
N$108: U5.7(INA) U6.12(ROUT1)
N$109: U5.6(OUTB) U6.11(DIN1)
N$110: C75.2 U6.2(V+)
N$111: C76.2 U6.6(V-)
N$112: C80.1 ISO_PULSE.1 U8.8(VCC2)
N$113: ISO_PULSE.2 U8.7(OUTA)
N$114: ISO_PULSE.3 U8.6(OUTB)
N$115: C80.2 ISO_PULSE.4 U8.5(GND2)
PORT_DTR: D51.2(A) RS1.4
PORT_RTS: D50.2(A) RS1.7
PORT_RX: RS1.2 U6.14(DOUT1)
PORT_TX: RS1.3 U6.13(RIN1)
REACT: JP11.1 U8.3(INB) ; also sheet 1
RS232_RXD: RX_EN.2 ; also sheet 1
RS232_TXD: TX_EN.2 ; also sheet 1
UART_RX: RX_EN.1 U5.2(OUTA)
UART_TX: TX_EN.1 U5.3(INB)
VCC_RS232: C71.1 C74.1 C77.1 JP14.1 U5.8(VCC2) U6.16(VCC) U7.5(OUT)
Unconnected: RS1.1 RS1.6 RS1.8 RS1.9 U6.7(DOUT2) U6.8(RIN2) U6.9(ROUT2) U6.10(DIN2) U7.4(NC/FB)

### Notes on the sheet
- Isolated RS232 Communication
- TPS70933
- ISO7321
- Act / React
- ISO7320
- TIDA-00839

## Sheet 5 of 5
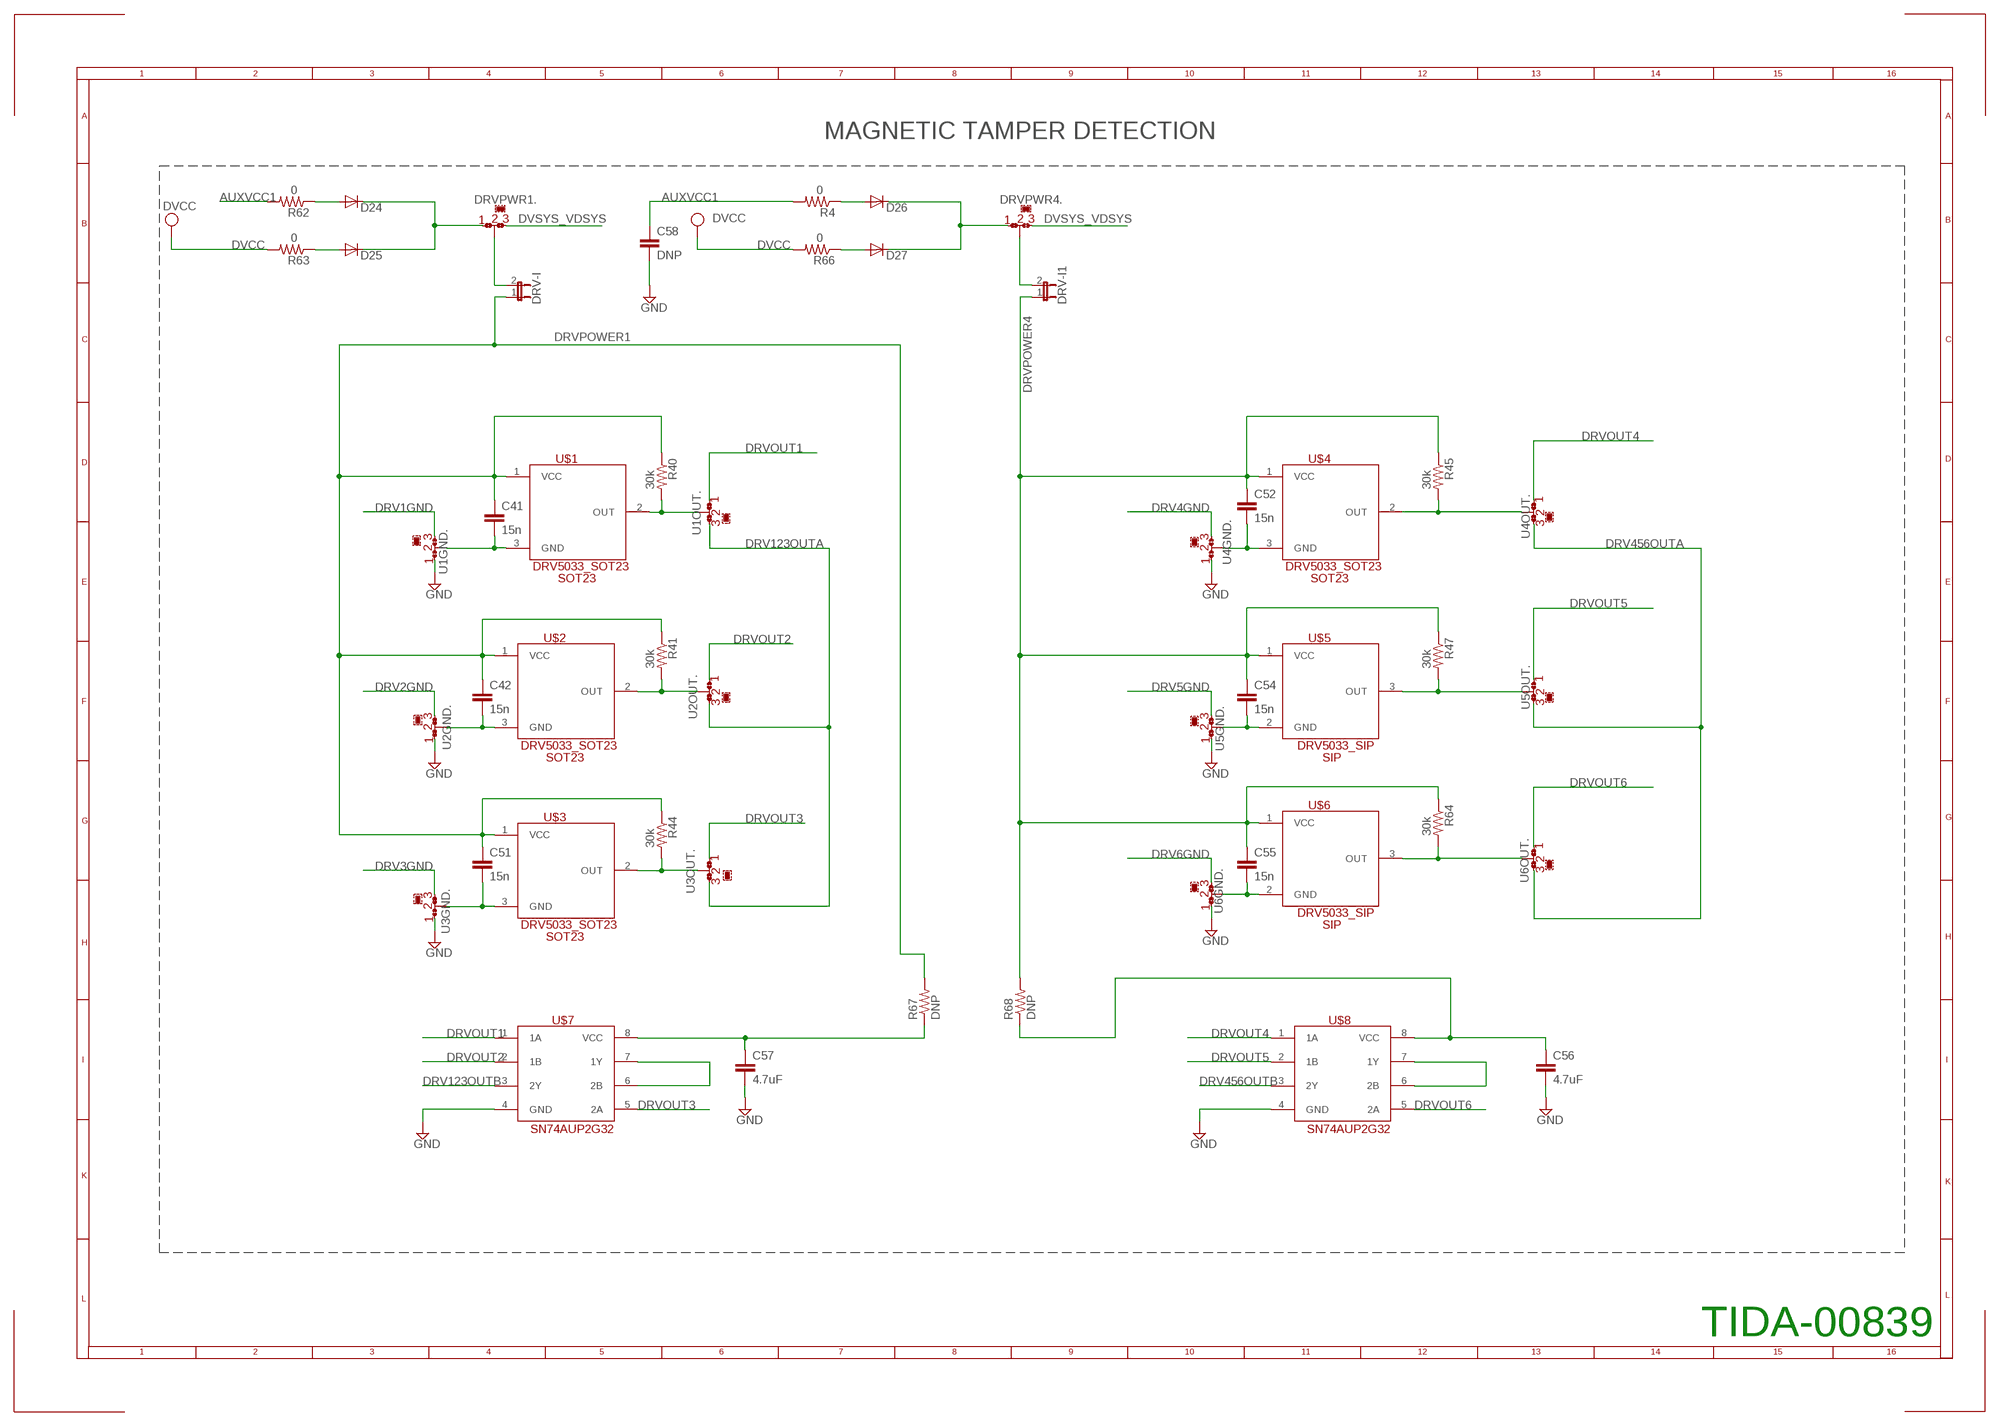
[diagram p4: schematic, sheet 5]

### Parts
C41  15n  C-EUC0805  [C0805]
C42  15n  C-EUC0805  [C0805]
C51  15n  C-EUC0805  [C0805]
C52  15n  C-EUC0805  [C0805]
C54  15n  C-EUC0805  [C0805]
C55  15n  C-EUC0805  [C0805]
C56  4.7uF  C-EUC0603  [C0603]
C57  4.7uF  C-EUC0603  [C0603]
C58  DNP  C-EUC0603  [C0603]
D24  PMLL4148  [SOD80C]
D25  PMLL4148  [SOD80C]
D26  PMLL4148  [SOD80C]
D27  PMLL4148  [SOD80C]
DRV-I  JP1E  [JP1]
DRV-I1  JP1E  [JP1]
DRVPWR1  0R-JUMPA  [A0R-JMP]
DRVPWR4  0R-JUMPA  [A0R-JMP]
R4  0  R-US_R0805  [R0805]
R40  30k  R-US_R0805  [R0805]
R41  30k  R-US_R0805  [R0805]
R44  30k  R-US_R0805  [R0805]
R45  30k  R-US_R0805  [R0805]
R47  30k  R-US_R0805  [R0805]
R62  0  R-US_R0805  [R0805]
R63  0  R-US_R0805  [R0805]
R64  30k  R-US_R0805  [R0805]
R66  0  R-US_R0805  [R0805]
R67  DNP  R-US_R0603  [R0603]
R68  DNP  R-US_R0603  [R0603]
U1GND  0R-JUMPA  [A0R-JMP]
U1OUT  0R-JUMPA  [A0R-JMP]
U2GND  0R-JUMPA  [A0R-JMP]
U2OUT  0R-JUMPA  [A0R-JMP]
U3GND  0R-JUMPA  [A0R-JMP]
U3OUT  0R-JUMPA  [A0R-JMP]
U4GND  0R-JUMPA  [A0R-JMP]
U4OUT  0R-JUMPA  [A0R-JMP]
U5GND  0R-JUMPA  [A0R-JMP]
U5OUT  0R-JUMPA  [A0R-JMP]
U6GND  0R-JUMPA  [A0R-JMP]
U6OUT  0R-JUMPA  [A0R-JMP]
U$1  DRV5033_SOT23  [SOT23]
U$2  DRV5033_SOT23  [SOT23]
U$3  DRV5033_SOT23  [SOT23]
U$4  DRV5033_SOT23  [SOT23]
U$5  DRV5033_SIP  [SIP]
U$6  DRV5033_SIP  [SIP]
U$7  SN74AUP2G32  [DCU]
U$8  SN74AUP2G32  [DCU]

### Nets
AUXVCC1: C58.1 R4.2 R62.2 ; also sheet 1
DRV1GND: U1GND.1 ; also sheet 1
DRV2GND: U2GND.1 ; also sheet 1
DRV3GND: U3GND.1 ; also sheet 1
DRV4GND: U4GND.1 ; also sheet 1
DRV5GND: U5GND.1 ; also sheet 1
DRV6GND: U6GND.1 ; also sheet 1
DRV123OUTA: U1OUT.1 U2OUT.1 U3OUT.1 ; also sheet 1
DRV123OUTB: U$7.3(2Y) ; also sheet 1
DRV456OUTA: U4OUT.1 U5OUT.1 U6OUT.1 ; also sheet 1
DRV456OUTB: U$8.3(2Y) ; also sheet 1
DRVOUT1: U1OUT.3 U$7.1(1A) ; also sheet 1
DRVOUT2: U2OUT.3 U$7.2(1B) ; also sheet 1
DRVOUT3: U3OUT.3 U$7.5(2A) ; also sheet 1
DRVOUT4: U4OUT.3 U$8.1(1A) ; also sheet 1
DRVOUT5: U5OUT.3 U$8.2(1B) ; also sheet 1
DRVOUT6: U6OUT.3 U$8.5(2A) ; also sheet 1
DRVPOWER1: C41.1 C42.1 C51.1 DRV-I.1 R40.1 R41.1 R44.1 R67.2 U$1.1(VCC) U$2.1(VCC) U$3.1(VCC)
DRVPOWER4: C52.1 C54.1 C55.1 DRV-I1.1 R45.1 R47.1 R64.1 R68.2 U$4.1(VCC) U$5.1(VCC) U$6.1(VCC)
DVCC: R63.2 R66.2 ; also sheet 1,3,4
DVSYS_VDSYS: DRVPWR1.1 DRVPWR4.1 ; also sheet 1
GND: C56.2 C57.2 C58.2 U1GND.3 U2GND.3 U3GND.3 U4GND.3 U5GND.3 U6GND.3 U$7.4(GND) U$8.4(GND) ; also sheet 1,2,3,4
N$1: D24.A R62.1
N$2: D25.A R63.1
N$9: D24.C D25.C DRVPWR1.3
N$11: C41.2 U1GND.2 U$1.3(GND)
N$12: C42.2 U2GND.2 U$2.3(GND)
N$22: C51.2 U3GND.2 U$3.3(GND)
N$24: C52.2 U4GND.2 U$4.3(GND)
N$26: C54.2 U5GND.2 U$5.2(GND)
N$28: C55.2 U6GND.2 U$6.2(GND)
N$35: DRV-I.2 DRVPWR1.2
N$41: R45.2 U4OUT.2 U$4.2(OUT)
N$43: R47.2 U5OUT.2 U$5.3(OUT)
N$45: U$7.6(2B) U$7.7(1Y)
N$49: D26.A R4.1
N$50: U$8.6(2B) U$8.7(1Y)
N$51: D27.A R66.1
N$52: D26.C D27.C DRVPWR4.3
N$53: DRV-I1.2 DRVPWR4.2
N$55: R64.2 U6OUT.2 U$6.3(OUT)
N$56: C57.1 R67.1 U$7.8(VCC)
N$58: C56.1 R68.1 U$8.8(VCC)
N$65: R40.2 U1OUT.2 U$1.2(OUT)
N$67: R41.2 U2OUT.2 U$2.2(OUT)
N$68: R44.2 U3OUT.2 U$3.2(OUT)

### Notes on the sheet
- MAGNETIC TAMPER DETECTION
- TIDA-00839

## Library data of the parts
ABTN3 ABTN4 DBTN1 DBTN2 RESET = electricalmeter:PB: OMRON SWITCH
C1-C21 C41 C42 C45 C47 C51 C52 C54 C55 C62 = rcl:C-EU: CAPACITOR, European symbol
C22-C38 C40 C43 C44 C48 C49 C53 C56-C58 C60 C61 = resistor:C-EU: CAPACITOR, European symbol
C39 C46 C50 = capacitor-wima:C: CAPACITOR
C63 = rcl:CPOL-US: POLARIZED CAPACITOR, American symbol; DIGIKEY: EEUEE2G100
C64 = rcl:C-US: CAPACITOR, American symbol; DIGIKEY: 06035C104KAT2A
C65 = rcl:CPOL-US: POLARIZED CAPACITOR, American symbol; DIGIKEY: 35ZL18MEFC5X7
C66 = rcl:CPOL-US: POLARIZED CAPACITOR, American symbol; DIGIKEY: 6.3ZL820MEFC8x16
C67 = rcl:C-US: CAPACITOR, American symbol; DIGIKEY: C3225X7R1E106M
C68 = rcl:C-US: CAPACITOR, American symbol; DIGIKEY: 08053C104KAT2A
C69 = rcl:C-EU: CAPACITOR, European symbol; DIGIKEY: 445-8047-1-ND
C70-C80 = rcl:C-EU: CAPACITOR, European symbol; DIGIKEY: 445-5956-1-ND
C102 = resistor:CPOL-EU: POLARIZED CAPACITOR, European symbol
D1-D16 D24-D43 = FE449x EVM:PMLL4148: DIODE
D17 D19 D21 = diode:1N4757A
D18 D20 D22 = diode:1N4007
D23 = diode:ZENER-DIODE: Z-Diode
D45 = diode:DIODE-: DIODE; DIGIKEY: US1J-E3/5AT
D46 = diode:DIODE-: DIODE; DIGIKEY: 1SMB5954BT3G
D47 = diode:DIODE-: DIODE; DIGIKEY: US1M-13-F
D48 = diode:DIODE-: DIODE; DIGIKEY: BAS20HT1G
D49 = diode:DIODE-: DIODE; DIGIKEY: B130LB-13-F
D50 D51 = zetex:D: DIODE; DIGIKEY: 1N4148WSFSCT-ND; MPN: CDSOD323-T05C; OC_FARNELL: 1824860; OC_NEWARK: 79R6078
DGND DVCC ISO_PULSE = custom_con-lstb:MA04-1: PIN HEADER; OC_FARNELL: unknown; OC_NEWARK: unknown
DRV-I DRV-I1 JP11 JP12 RX_EN TX_EN = custom_jumper:JP1E: JUMPER
DRVPWR1 DRVPWR4 U1GND U1OUT U2GND U2OUT U3GND U3OUT U4GND U4OUT U5GND U5OUT U6GND U6OUT = jump-0r-smd:0R-JUMP: SMD 0R 0805 Jumper
I1+ I1- I2+ I2- I3+ I3- IN+ IN- LINE1-LINE3 NEUTRAL = testpad:TP: Test pad
JP3-JP10 = custom_jumper:JP2E: JUMPER
JP14 = jumper:JP1E: JUMPER; DIGIKEY: 609-4434-ND
JTAG = con-ml:ML14: HARTING; OC_FARNELL: unknown; OC_NEWARK: unknown
L1 L3 L5 L6 = FE449x EVM:EXCELSA39: INDUCTOR
L7 = rcl:L-US: INDUCTOR, American symbol
LCD1 = Personal:TI_160SEG_LCD
LED1-LED6 LED_ACT LED_REACT = led:LED: LED
MSP430F67791A = Personal:MSP430F6779AIPEU: MSP430F6779IPEU
R1-R3 = varistor:S20K275: VARISTOR
R4 R20-R23 R35 R37 R38 R40 R41 R44 R45 R47 R62-R64 R66 R92-R95 = resistor:R-US_: RESISTOR, American symbol
R5-R19 R24-R34 R36 R39 R65 = _MSP430:RES
R42 R43 R46 R48-R61 = resistor:R-EU_: RESISTOR, European symbol
R67 R68 R96-R98 R/L7-R/L14 = rcl:R-US_: RESISTOR, American symbol
R104 = rcl:R-US_: RESISTOR, American symbol; DIGIKEY: CRCW06032K87FKEA
R105 = rcl:R-US_: RESISTOR, American symbol; DIGIKEY: CRCW060330K1FKEA
R106 = rcl:R-US_: RESISTOR, American symbol; DIGIKEY: CRCW060376K8FKEA
R107 = rcl:R-US_: RESISTOR, American symbol; DIGIKEY: CRCW060310R0FKEA
R108 = rcl:R-US_: RESISTOR, American symbol; DIGIKEY: CRCW06032K00JNEA
RS1 = con-subd:F09VP: SUB-D; DIGIKEY: A32119-ND; OC_FARNELL: unknown; OC_NEWARK: unknown
RTC = SparkFun:M02: Header 2
SV1 = jumper:JP3Q: JUMPER
T1 = RencoTransformer:CUSTOMTRANS; TI: CustomTrans
TVS1-TVS4 = FE449x EVM:SMAJ5.0CA
U3 = TPS54060:TPS54060_DGQ_10; DATASHEETURL: http://www.ti.com/lit/gpn/TPS54060; DESCRIPTION: 3.5V to 60V Input, 0.5A Step-Down Converter with Eco-Mode; FAMILY_NAME: STEP-DOWN REGULATOR; GENERIC_PART_NUMBER: TPS54060; INDUSTRY_STD_PKG_TYPE: MSOP-PowerPAD; MANUFACTURER: Texas Instruments; MANUFACTURER_PART_NUMBER: tps54060_dgq_10; PACKAGE_DESIGNATOR: DGQ; PIN_COUNT: 10; VENDOR: Texas Instruments
U4 = UCC28910:UCC28910D; DIGIKEY: UCC28910D
U5 = Texas Instruments_By_element14_Batch_1:ISO7421D: Low-Power Dual Digital Isolators; DIGIKEY: 296-25187-5-ND; MPN: ISO7421D; OC_FARNELL: -; OC_NEWARK: 33R2484; PACKAGE: SOIC-8; SUPPLIER: Texas Instruments
U6 = Texas Instruments_By_element14_Batch_1:TRS3232EQPWRQ1: RS-232 LINE DRIVER/RECEIVER; DIGIKEY: 296-24863-1-ND; MPN: TRS3232EQPWRQ1; OC_FARNELL: -; OC_NEWARK: 09R6724; PACKAGE: TSSOP-16; SUPPLIER: Texas Instruments
U7 = Texas Instruments_By_element14_Batch_1:TPS76333DBVT: Low Power 150mA Low Dropout Linear Regulator; DIGIKEY: 296-11021-1-ND; MPN: TPS76333DBVT; OC_FARNELL: 8461376; OC_NEWARK: 96C8605; PACKAGE: SOT-23-5; SUPPLIER: Texas Instruments
U8 = TIiso:ISO7420_D_8; DATASHEETURL: http://www.ti.com/lit/gpn/ISO7420; DESCRIPTION: Low Power Dual Channel Isolators; FAMILY_NAME: ISOLATOR; GENERIC_PART_NUMBER: ISO7420; INDUSTRY_STD_PKG_TYPE: SOIC; MANUFACTURER: Texas Instruments; MANUFACTURER_PART_NUMBER: iso7420_d_8; PACKAGE_DESIGNATOR: D; PIN_COUNT: 8; VENDOR: Texas Instruments
U$1-U$4 = DRVlibrary:DRV5033_SOT23
U$5 U$6 = DRVlibrary:DRV5033_SIP
U$7 U$8 = SN74AUP2G32:SN74AUP2G32
XT1 = F20xx PIR Demo & Eval:CM200T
